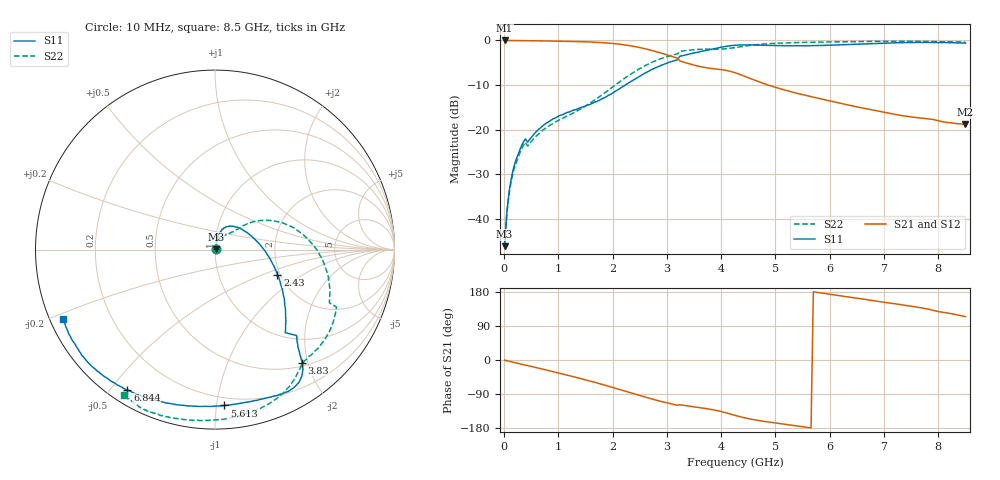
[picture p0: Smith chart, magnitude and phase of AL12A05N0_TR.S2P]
!AVX CORPORATION
!PART NUMBER AL12A05N0_TR
!DESCRIPTION: AIR CORE INDUCTOR, 5nH, 2 TURNS
!Agilent Technologies,E5071C,MY46102230,A.09.54
!Date: Mon Sep 03 15:49:53 2012
!Data & Calibration Information:
!Freq	S11:SOLT2(ON)	S21:SOLT2(ON)	S12:SOLT2(ON)	S22:SOLT2(ON)
# Hz S RI R 50
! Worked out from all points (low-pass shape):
!   201 points, 10 MHz to 8.5 GHz, reference 50 ohm
!   highest |S21| = -0.04 dB at 10 MHz (marker M1); lowest = -18.9 dB at 8.5 GHz (marker M2)
!   |S21| within 3 dB of the highest: start of sweep to 2.942 GHz
!   lowest |S11| = -46.1 dB at 10 MHz (marker M3), VSWR 1.01, Z = 50.5 + j0.188 ohm
!   |S11| at or under -10 dB: start of sweep to 2.238 GHz
!   |S22| runs from -45.6 to -0.2 dB; largest |S21 - S12| = 0.013
!   S11 on the Smith chart (normalised r, x): 10 MHz: 1.01, +0.00; 2.43 GHz: 1.93, -0.62; 3.83 GHz: 0.56, -1.91; 5.613 GHz: 0.15, -1.05; 6.844 GHz: 0.05, -0.55; 8.5 GHz: 0.04, -0.22
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1e7  0.00457 0.00186  0.9954 -0.00665  0.9914 0.0054  0.00489 0.00191
5.245e7  0.00469 0.011  0.9944 -0.0322  0.9983 -0.0331  0.00501 0.0107
9.49e7  0.00562 0.0199  0.9924 -0.0578  0.9936 -0.057  0.00672 0.0182
1.3735e8  0.00651 0.0285  0.9902 -0.0831  0.9911 -0.0824  0.00846 0.0261
2.2225e8  0.00915 0.0453  0.9833 -0.1332  0.9854 -0.1339  0.0131 0.0405
3.496e8  0.016 0.0693  0.9678 -0.2074  0.9695 -0.2081  0.023 0.0612
4.345e8  0.0164 0.0704  0.9567 -0.2515  0.9578 -0.2529  0.0282 0.0588
9.0145e8  0.0506 0.1213  0.8423 -0.4992  0.8426 -0.5005  0.0761 0.0889
1.4533e9  0.1317 0.1211  0.6114 -0.7433  0.6114 -0.7443  0.131 0.117
2.00515e9  0.2568 0.0197  0.2748 -0.8785  0.2741 -0.8794  0.2531 0.1624
2.42965e9  0.3477 -0.139  -0.0107 -0.8454  -0.0109 -0.8454  0.4378 0.1215
2.85415e9  0.3922 -0.3284  -0.2245 -0.6957  -0.2251 -0.6957  0.6062 -0.0735
3.19375e9  0.3912 -0.4624  -0.3099 -0.5507  -0.3102 -0.5508  0.6376 -0.2967
3.2362e9  0.4541 -0.4788  -0.2775 -0.5186  -0.2779 -0.5184  0.6771 -0.3203
3.8305e9  0.4856 -0.6294  -0.3154 -0.3668  -0.3154 -0.3668  0.5382 -0.5855
4.255e9  0.4571 -0.751  -0.3593 -0.2414  -0.3598 -0.2413  0.4593 -0.6886
4.9342e9  0.2864 -0.8266  -0.2955 -0.0798  -0.2958 -0.0795  0.2491 -0.8875
5.6134e9  0.0524 -0.8682  -0.237 -0.00668  -0.2371 -0.0066  0.00497 -0.9488
5.6983e9  0.0183 -0.8711  -0.2306 0.000594  -0.2307 0.000743  -0.0246 -0.9495
6.84445e9  -0.488 -0.7822  -0.1487 0.0667  -0.1487 0.0668  -0.3 -0.9257
7.09915e9  -0.5741 -0.7358  -0.1319 0.0752  -0.1319 0.0752  -0.3435 -0.9117
8.5e9  -0.8448 -0.3867  -0.0472 0.1038  -0.0472 0.1036  -0.5067 -0.8102
